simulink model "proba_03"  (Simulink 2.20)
settings: Solver=ode45  StartTime=0.0  StopTime=100.0  FixedStep=1  RelTol=1e-3  AbsTol=1e-6
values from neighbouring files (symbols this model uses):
  q0 = P+q2    [DPIDrc_S.m]    (also in PID01.m; ab2pq.m = 1.0/sum(B))
  q1 = -P+P*(h/I)-2*q2    [DPIDrc_S.m]    (also in PID01.m)
  q2 = P*(D/h)    [DPIDrc_S.m]    (also in PID01.m)

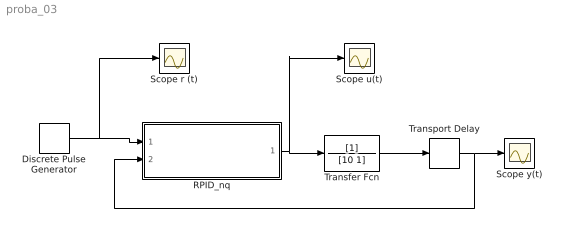
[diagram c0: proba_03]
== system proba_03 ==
  Discrete Pulse Generator : DiscretePulseGenerator  Amplitude=1  Period=100  PulseWidth=100  PhaseDelay=1  SampleTime=2
  RPID_nq : Subsystem  mask(discret PID regulator){P=1, I=5, D=1, h=1}
      mask prompts: P ":"; I "I [s]:"; D "D [s]:"; h "h [s]:"
      mask help: Presmiata koeficientitr za diskreten PID regulatorpri zadadeni: P, I, D - vremenkonstantite na neprekasnatia; h - stapka na diskretizacia;
      mask init:
      | %  Documentation
      |             P=@1;I=@2;D=@3;h=@4;
      | [q0,q1,q2]=pid01(P,I,D,h);
  Scope r (t) : Scope
  Scope u(t) : Scope
  Scope y(t) : Scope
  Transfer Fcn : TransferFcn  Numerator=[1]  Denominator=[10 1]
  Transport Delay : TransportDelay  DelayTime=2  InitialInput=0  BufferSize=1024
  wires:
  Discrete Pulse Generator/1 -> Scope r (t)/1, RPID_nq/1(In1)
  Transfer Fcn/1 -> Transport Delay/1
  RPID_nq/1(Out1) -> Transfer Fcn/1, Scope u(t)/1
  Transport Delay/1 -> Scope y(t)/1, RPID_nq/2(In2)

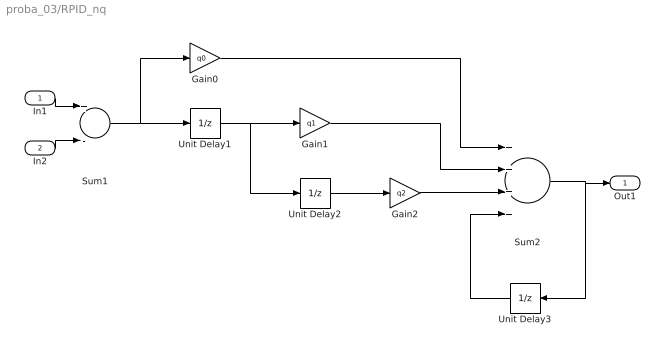
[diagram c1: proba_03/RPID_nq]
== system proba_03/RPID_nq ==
  In1 : Inport  Port=1  PortWidth=-1  SampleTime=-1
  In2 : Inport  Port=2  PortWidth=-1  SampleTime=-1
  Gain0 : Gain  Description=GAIN 0  Gain=q0
  Gain1 : Gain  Description=Gain 1  Gain=q1
  Gain2 : Gain  Gain=q2
  Sum1 : Sum  Inputs=+-
  Sum2 : Sum  Inputs=++++
  Unit Delay1 : UnitDelay  Description=Gain 0  X0=0  SampleTime=1
  Unit Delay2 : UnitDelay  Description=Gain 1  X0=0  SampleTime=1
  Unit Delay3 : UnitDelay  Orientation=left  X0=0  SampleTime=1
  Out1 : Outport  Port=1  InitialOutput=0
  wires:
  In2/1 -> Sum1/2
  In1/1 -> Sum1/1
  Unit Delay3/1 -> Sum2/4
  Sum2/1 -> Out1/1, Unit Delay3/1
  Gain2/1 -> Sum2/3
  Gain1/1 -> Sum2/2
  Unit Delay2/1 -> Gain2/1
  Unit Delay1/1 -> Unit Delay2/1, Gain1/1
  Gain0/1 -> Sum2/1
  Sum1/1 -> Gain0/1, Unit Delay1/1
